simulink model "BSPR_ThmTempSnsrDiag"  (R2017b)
settings: Solver=FixedStepDiscrete  StartTime=0.0  StopTime=10.0  FixedStep=0.02  RelTol=1e-3  EnableMultiTasking=on
undefined symbols (not defined in the file): BCCR_cntClntTempDiag_CW, bin2dec, BSPR_tClntDsTOvrTemp_C, BSPR_tClntUsTOvrTemp_C, BSPR_tiClntDsTElecMax_C, BSPR_tiClntDsTElecMin_C, BSPR_tiClntDsTJit_C, BSPR_tiClntDsTOvrTemp_C, BSPR_tiClntDsTVld_C, BSPR_tiClntUsTElecMax_C, BSPR_tiClntUsTElecMin_C, BSPR_tiClntUsTJit_C, BSPR_tiClntUsTOvrTemp_C, BSPR_tiClntUsTVld_C, BSPR_uClntDsTElecMax_C, BSPR_uClntDsTElecMin_C, BSPR_uClntDsTJitDiff_C, BSPR_uClntUsTElecMax_C, BSPR_uClntUsTElecMin_C, BSPR_uClntUsTJitDiff_C
libraries: simulink x64
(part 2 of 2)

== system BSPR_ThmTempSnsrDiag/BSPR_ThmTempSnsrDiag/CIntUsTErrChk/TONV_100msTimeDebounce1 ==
  note: Turn On Delay Time Deboune
  u : Inport
  T : Inport  Port=2
  Add : Sum
  Constant1 : Constant  Value=0  OutDataTypeStr=single
  Constant2 : Constant  OutDataTypeStr=uint8
  Constant3 : Constant  Value=0  OutDataTypeStr=uint8
  Constant4 : Constant  Value=0.1  OutDataTypeStr=single
  Delay : Delay  DelayLength=1  InitialCondition=0
  MinMax : MinMax  Inputs=2
  Product : Product  OutMin=[0]  OutMax=[65535]  OutDataTypeStr=single
  Relational Operator : RelationalOperator  Operator=>  OutDataTypeStr=boolean  RndMeth=Simplest
  Switch : Switch  Criteria=u2 ~= 0
  Switch1 : Switch  Criteria=u2 ~= 0
  y : Outport
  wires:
  MinMax/1 -> Add/2
  T/1 -> Relational Operator/2, MinMax/1
  Relational Operator/1 -> y/1
  Delay/1 -> MinMax/2
  Switch/1 -> Add/1
  Product/1 -> Delay/1, Relational Operator/1
  Add/1 -> Product/2
  Constant1/1 -> Switch/3
  Constant4/1 -> Switch/1
  u/1 -> Switch/2, Switch1/2
  Constant2/1 -> Switch1/1
  Constant3/1 -> Switch1/3
  Switch1/1 -> Product/1

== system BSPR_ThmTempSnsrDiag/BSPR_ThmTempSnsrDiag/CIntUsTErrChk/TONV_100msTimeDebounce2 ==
  note: Turn On Delay Time Deboune
  u : Inport
  T : Inport  Port=2
  Add : Sum
  Constant1 : Constant  Value=0  OutDataTypeStr=single
  Constant2 : Constant  OutDataTypeStr=uint8
  Constant3 : Constant  Value=0  OutDataTypeStr=uint8
  Constant4 : Constant  Value=0.1  OutDataTypeStr=single
  Delay : Delay  DelayLength=1  InitialCondition=0
  MinMax : MinMax  Inputs=2
  Product : Product  OutMin=[0]  OutMax=[65535]  OutDataTypeStr=single
  Relational Operator : RelationalOperator  Operator=>  OutDataTypeStr=boolean  RndMeth=Simplest
  Switch : Switch  Criteria=u2 ~= 0
  Switch1 : Switch  Criteria=u2 ~= 0
  y : Outport
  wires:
  MinMax/1 -> Add/2
  T/1 -> Relational Operator/2, MinMax/1
  Relational Operator/1 -> y/1
  Delay/1 -> MinMax/2
  Switch/1 -> Add/1
  Product/1 -> Delay/1, Relational Operator/1
  Add/1 -> Product/2
  Constant1/1 -> Switch/3
  Constant4/1 -> Switch/1
  u/1 -> Switch/2, Switch1/2
  Constant2/1 -> Switch1/1
  Constant3/1 -> Switch1/3
  Switch1/1 -> Product/1

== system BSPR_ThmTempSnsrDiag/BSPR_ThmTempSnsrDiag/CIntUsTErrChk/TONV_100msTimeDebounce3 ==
  note: Turn On Delay Time Deboune
  u : Inport
  T : Inport  Port=2
  Add : Sum
  Constant1 : Constant  Value=0  OutDataTypeStr=single
  Constant2 : Constant  OutDataTypeStr=uint8
  Constant3 : Constant  Value=0  OutDataTypeStr=uint8
  Constant4 : Constant  Value=0.1  OutDataTypeStr=single
  Delay : Delay  DelayLength=1  InitialCondition=0
  MinMax : MinMax  Inputs=2
  Product : Product  OutMin=[0]  OutMax=[65535]  OutDataTypeStr=single
  Relational Operator : RelationalOperator  Operator=>  OutDataTypeStr=boolean  RndMeth=Simplest
  Switch : Switch  Criteria=u2 ~= 0
  Switch1 : Switch  Criteria=u2 ~= 0
  y : Outport
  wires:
  Switch1/1 -> Product/1
  Constant3/1 -> Switch1/3
  Constant2/1 -> Switch1/1
  u/1 -> Switch1/2, Switch/2
  Constant4/1 -> Switch/1
  Constant1/1 -> Switch/3
  Add/1 -> Product/2
  Product/1 -> Relational Operator/1, Delay/1
  Switch/1 -> Add/1
  Delay/1 -> MinMax/2
  Relational Operator/1 -> y/1
  T/1 -> MinMax/1, Relational Operator/2
  MinMax/1 -> Add/2

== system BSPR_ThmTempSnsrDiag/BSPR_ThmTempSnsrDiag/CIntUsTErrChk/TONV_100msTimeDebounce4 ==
  note: Turn On Delay Time Deboune
  u : Inport
  T : Inport  Port=2
  Add : Sum
  Constant1 : Constant  Value=0  OutDataTypeStr=single
  Constant2 : Constant  OutDataTypeStr=uint8
  Constant3 : Constant  Value=0  OutDataTypeStr=uint8
  Constant4 : Constant  Value=0.1  OutDataTypeStr=single
  Delay : Delay  DelayLength=1  InitialCondition=0
  MinMax : MinMax  Inputs=2
  Product : Product  OutMin=[0]  OutMax=[65535]  OutDataTypeStr=single
  Relational Operator : RelationalOperator  Operator=>  OutDataTypeStr=boolean  RndMeth=Simplest
  Switch : Switch  Criteria=u2 ~= 0
  Switch1 : Switch  Criteria=u2 ~= 0
  y : Outport
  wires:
  Switch1/1 -> Product/1
  Constant3/1 -> Switch1/3
  Constant2/1 -> Switch1/1
  u/1 -> Switch1/2, Switch/2
  Constant4/1 -> Switch/1
  Constant1/1 -> Switch/3
  Add/1 -> Product/2
  Product/1 -> Relational Operator/1, Delay/1
  Switch/1 -> Add/1
  Delay/1 -> MinMax/2
  Relational Operator/1 -> y/1
  T/1 -> MinMax/1, Relational Operator/2
  MinMax/1 -> Add/2

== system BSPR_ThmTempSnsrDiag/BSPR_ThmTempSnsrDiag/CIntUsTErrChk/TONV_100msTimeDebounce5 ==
  note: Turn On Delay Time Deboune
  u : Inport
  T : Inport  Port=2
  Add : Sum
  Constant1 : Constant  Value=0  OutDataTypeStr=single
  Constant2 : Constant  OutDataTypeStr=uint8
  Constant3 : Constant  Value=0  OutDataTypeStr=uint8
  Constant4 : Constant  Value=0.1  OutDataTypeStr=single
  Delay : Delay  DelayLength=1  InitialCondition=0
  MinMax : MinMax  Inputs=2
  Product : Product  OutMin=[0]  OutMax=[65535]  OutDataTypeStr=single
  Relational Operator : RelationalOperator  Operator=>  OutDataTypeStr=boolean  RndMeth=Simplest
  Switch : Switch  Criteria=u2 ~= 0
  Switch1 : Switch  Criteria=u2 ~= 0
  y : Outport
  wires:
  MinMax/1 -> Add/2
  T/1 -> Relational Operator/2, MinMax/1
  Relational Operator/1 -> y/1
  Delay/1 -> MinMax/2
  Switch/1 -> Add/1
  Product/1 -> Delay/1, Relational Operator/1
  Add/1 -> Product/2
  Constant1/1 -> Switch/3
  Constant4/1 -> Switch/1
  u/1 -> Switch/2, Switch1/2
  Constant2/1 -> Switch1/1
  Constant3/1 -> Switch1/3
  Switch1/1 -> Product/1

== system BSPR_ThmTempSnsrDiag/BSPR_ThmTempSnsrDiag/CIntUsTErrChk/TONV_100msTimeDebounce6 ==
  note: Turn On Delay Time Deboune
  u : Inport
  T : Inport  Port=2
  Add : Sum
  Constant1 : Constant  Value=0  OutDataTypeStr=single
  Constant2 : Constant  OutDataTypeStr=uint8
  Constant3 : Constant  Value=0  OutDataTypeStr=uint8
  Constant4 : Constant  Value=0.1  OutDataTypeStr=single
  Delay : Delay  DelayLength=1  InitialCondition=0
  MinMax : MinMax  Inputs=2
  Product : Product  OutMin=[0]  OutMax=[65535]  OutDataTypeStr=single
  Relational Operator : RelationalOperator  Operator=>  OutDataTypeStr=boolean  RndMeth=Simplest
  Switch : Switch  Criteria=u2 ~= 0
  Switch1 : Switch  Criteria=u2 ~= 0
  y : Outport
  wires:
  MinMax/1 -> Add/2
  T/1 -> Relational Operator/2, MinMax/1
  Relational Operator/1 -> y/1
  Delay/1 -> MinMax/2
  Switch/1 -> Add/1
  Product/1 -> Delay/1, Relational Operator/1
  Add/1 -> Product/2
  Constant1/1 -> Switch/3
  Constant4/1 -> Switch/1
  u/1 -> Switch/2, Switch1/2
  Constant2/1 -> Switch1/1
  Constant3/1 -> Switch1/3
  Switch1/1 -> Product/1

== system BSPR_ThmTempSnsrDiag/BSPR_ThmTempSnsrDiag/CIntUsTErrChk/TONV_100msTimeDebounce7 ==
  note: Turn On Delay Time Deboune
  u : Inport
  T : Inport  Port=2
  Add : Sum
  Constant1 : Constant  Value=0  OutDataTypeStr=single
  Constant2 : Constant  OutDataTypeStr=uint8
  Constant3 : Constant  Value=0  OutDataTypeStr=uint8
  Constant4 : Constant  Value=0.1  OutDataTypeStr=single
  Delay : Delay  DelayLength=1  InitialCondition=0
  MinMax : MinMax  Inputs=2
  Product : Product  OutMin=[0]  OutMax=[65535]  OutDataTypeStr=single
  Relational Operator : RelationalOperator  Operator=>  OutDataTypeStr=boolean  RndMeth=Simplest
  Switch : Switch  Criteria=u2 ~= 0
  Switch1 : Switch  Criteria=u2 ~= 0
  y : Outport
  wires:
  Switch1/1 -> Product/1
  Constant3/1 -> Switch1/3
  Constant2/1 -> Switch1/1
  u/1 -> Switch1/2, Switch/2
  Constant4/1 -> Switch/1
  Constant1/1 -> Switch/3
  Add/1 -> Product/2
  Product/1 -> Relational Operator/1, Delay/1
  Switch/1 -> Add/1
  Delay/1 -> MinMax/2
  Relational Operator/1 -> y/1
  T/1 -> MinMax/1, Relational Operator/2
  MinMax/1 -> Add/2
